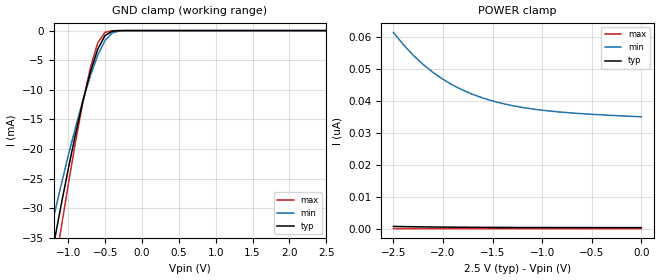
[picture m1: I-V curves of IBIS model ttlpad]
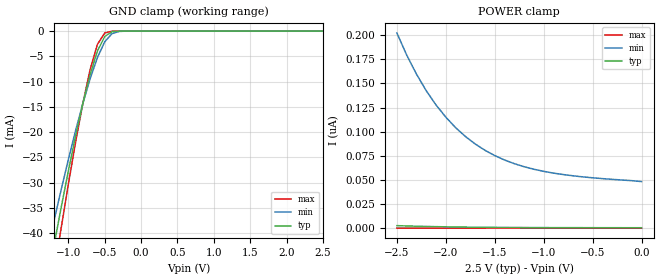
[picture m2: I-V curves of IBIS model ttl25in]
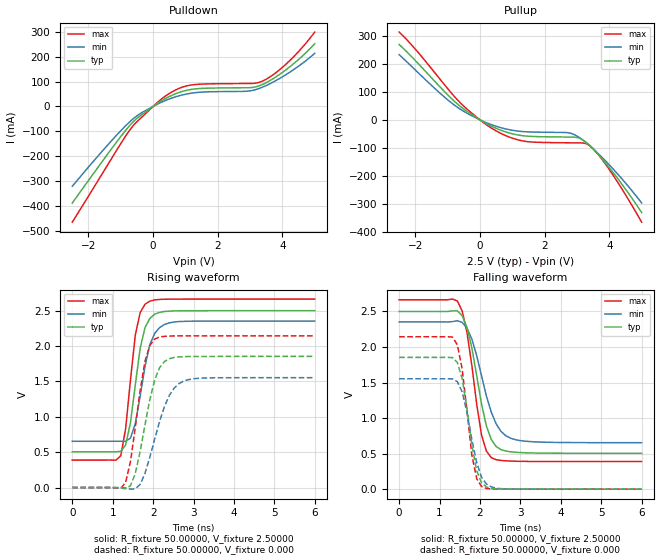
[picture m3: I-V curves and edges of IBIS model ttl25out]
| IBIS file idt45t9070.ibs created by s2ibis2 version 1.2
| North Carolina State University Electronics Research Laboratory  1995
[IBIS ver]   3.2
[File name]   idt45t9070.ibs
[File Rev]   1.0
[Date]   Friday, November 09, 2001
[Source]   Integrated Device Technology, Inc.
[Notes]
[Disclaimer] Integrated Device Technology, Inc. ("IDT") hereby grants the
   user of this IBIS model a non-exclusive, nontransferable
   license to use this IBIS model under the following terms. The
   user is granted this license only to use the IBIS model and is
   not granted rights to sell, copy (except as needed to run the
   IBIS model), rent, lease or sub-license the IBIS model in
   whole or in part, or in modified form to anyone. The User may
   modify the IBIS model to suit its specific applications, but
   rights to derivative works and such modifications shall belong
   to IDT. This IBIS model is provided on an AS IS" basis and IDT
   makes absolutely no warranty with respect to the information
   contained herein. IDT DISCLAIMS AND CUSTOMER WAIVES ALL
   WARRANTIES, EXPRESS AND IMPLIED, INCLUDING WARRANTIES OF
   MERCHANTABILITY AND FITNESS FOR A PARTICULAR PURPOSE. THE
   ENTIRE RISK AS TO QUALITY AND PERFORMANCE IS WITH THE USER
   ACCORDINGLY, IN NO EVENT SHALL IDT BE LIABLE FOR ANY DIRECT OR
   INDIRECT DAMAGES, WHETHER IN CONTRACT OR TORT, INCLUDING ANY
   LOST PROFITS OR OTHER INCIDENTAL, CONSEQUENTIAL, EXEMPLARY, OR
   PUNITIVE DAMAGES ARISING OUT OF THE USE OR APPLICATION OF THE
   IBIS model. Further, IDT reserves the right to make changes
   without notice to any product herein to improve reliability,
   function, or design. IDT does not convey any license under
   patent rights or any other intellectual property rights,
   including those of third parties. IDT is not obligated to
   provide maintenance or support for the licensed IBIS model.
[Copyright]   Copyright 2001, Integrated Device Technology, Inc. all rights
   reserved
|   Component idt45t9070
[Component]   idt45t9070
[Manufacturer]   Integrated Device Technology
|Package   PA48
[Package]
| variable   typ   min   max
R_pkg   6.00000m   6.00000m   6.00000m
L_pkg   3.00000nH   3.00000nH   3.00000nH
C_pkg   0.20000pF   0.20000pF   0.20000pF
[Pin]  signal_name   model_name   R_pin   L_pin   C_pin
1   gl   ttlpad
2   vdd   POWER
3   vdd   POWER
4   gnd   GND
5   gnd   GND
6   g1x   ttlpad
7   vddq   POWER
8   q2   ttl25out
9   q1   ttl25out
10   gnd   GND
11   vddq   POWER
12   gnd   GND
13   a   ttl25in
14   vddq   POWER
15   gnd   GND
16   q10   ttl25out
17   q9   ttl25out
18   vddq   POWER
19   g2x   ttlpad
20   gnd   GND
21   gnd   GND
22   vdd   POWER
23   vdd   POWER
24   NC   NC
25   NC   NC
26   gnd   GND
27   vddq   POWER
28   gnd   GND
29   gnd   GND
30   vddq   POWER
31   vddq   POWER
32   q8   ttl25out
33   q7   ttl25out
34   gnd   GND
35   vddq   POWER
36   q6   ttl25out
37   q5   ttl25out
38   vddq   POWER
39   gnd   GND
40   q4   ttl25out
41   q3   ttl25out
42   vddq   POWER
43   gnd   GND
44   gnd   GND
45   gnd   GND
46   vddq   POWER
47   vddq   POWER
48   gnd   GND
[Pin Mapping]  pulldown_ref   pullup_ref   gnd_clamp_ref   power_clamp_ref
1   gnd   vdd
2   NC   vdd
3   NC   vdd
4   gnd   NC
5   gnd   NC
6   gnd   vdd
7   NC   vddq
8   gnd   vddq
9   gnd   vddq
10   gnd   NC
11   NC   vddq
12   gnd   NC
13   gnd   vdd
14   NC   vddq
15   gnd   NC
16   gnd   vddq
17   gnd   vddq
18   NC   vddq
19   gnd   vdd
20   gnd   NC
21   gnd   NC
22   NC   vdd
23   NC   vdd
24   NC   NC
25   NC   NC
26   gnd   NC
27   NC   vddq
28   gnd   NC
29   gnd   NC
30   NC   vddq
31   NC   vddq
32   gnd   vddq
33   gnd   vddq
34   gnd   NC
35   NC   vddq
36   gnd   vddq
37   gnd   vddq
38   NC   vddq
39   gnd   NC
40   gnd   vddq
41   gnd   vddq
42   NC   vddq
43   gnd   NC
44   gnd   NC
45   gnd   NC
46   NC   vddq
47   NC   vddq
48   gnd   NC
| Models and submodels in the file (3): ttlpad (Input), ttl25in (Input), ttl25out (Output)
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|   Model ttlpad
[Model]   ttlpad
Model_type   Input
Polarity   Non-Inverting
Vinl =  0.70000V
Vinh =  1.70000V
Vmeas =  1.25000V
C_comp   5.00000pF   5.00000pF   5.00000pF
[Temperature Range]   45.00000   0.14000k   -30.00000
[Voltage Range]   2.50000V   2.30000V   2.70000V
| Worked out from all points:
|   GND clamp passes 1 mA (typ) near -0.51 V on its own axis
[GND_clamp]
| voltage   I(typ)   I(min)   I(max)
-2.5V     -129.2mA   -109.1mA   -150.6mA
-1.3V     -43.01mA   -37.08mA   -49.74mA
-1.2V     -36.24mA   -31.57mA   -41.59mA
-1.1V     -29.66mA   -26.23mA   -33.63mA
-900mV    -17.36mA   -16.23mA   -18.68mA
-800mV    -11.85mA   -11.7mA    -12mA
-700mV    -6.996mA   -7.615mA   -6.253mA
-600mV    -3.137mA   -4.151mA   -2.071mA
-500mV    -815.1uA   -1.634mA   -278.8uA
-400mV    -95.37uA   -373.7uA   -14.75uA
-300mV    -5.658uA   -48.78uA   -281.7nA
2.5V      324.7pA    35.28nA    828.2fA
[POWER_clamp]
| voltage   I(typ)   I(min)   I(max)
-2.5V     698.6pA    61.39nA    2.05pA
-2.4V     644.6pA    57.56nA    1.88pA
-2.3V     597.5pA    54.23nA    1.737pA
-2.2V     556.7pA    51.34nA    1.611pA
-2.1V     521.4pA    48.85nA    1.499pA
-1.9V     465pA      44.88nA    1.333pA
-1.8V     442.7pA    43.32nA    1.256pA
-1.6V     407.7pA    40.88nA    1.155pA
-1.3V     373.1pA    38.48nA    1.037pA
-1V       352.5pA    37.05nA    965.9fA
-600mV    337.2pA    35.97nA    899.5fA
0V        324.7pA    34.99nA    849.9fA
|   Model ttl25in
[Model]   ttl25in
Model_type   Input
Polarity   Non-Inverting
Vinl =  0.70000V
Vinh =  1.70000V
Vmeas =  1.25000V
C_comp   5.00000pF   5.00000pF   5.00000pF
[Temperature Range]   45.00000   0.14000k   -30.00000
[Voltage Range]   2.50000V   2.30000V   2.70000V
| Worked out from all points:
|   GND clamp passes 1 mA (typ) near -0.49 V on its own axis
[GND_clamp]
| voltage   I(typ)   I(min)   I(max)
-2.5V     -150.1mA   -128.5mA   -173mA
-1.3V     -50.47mA   -44.23mA   -57.51mA
-1.2V     -42.64mA   -37.76mA   -48.2mA
-1.1V     -35.02mA   -31.48mA   -39.1mA
-900mV    -20.73mA   -19.68mA   -21.96mA
-800mV    -14.28mA   -14.3mA    -14.26mA
-700mV    -8.553mA   -9.407mA   -7.567mA
-600mV    -3.939mA   -5.223mA   -2.609mA
-500mV    -1.074mA   -2.122mA   -375.8uA
-400mV    -131.3uA   -507.1uA   -20.31uA
-300mV    -7.825uA   -67.79uA   -384.6nA
2.5V      443.6pA    49.9nA     1.135pA
[POWER_clamp]
| voltage   I(typ)   I(min)   I(max)
-2.5V     2.616nA    202.4nA    8.153pA
-2.4V     2.294nA    179.5nA    7.17pA
-2.3V     2.014nA    159.7nA    6.305pA
-2.2V     1.772nA    142.5nA    5.573pA
-2.1V     1.564nA    127.7nA    4.925pA
-1.9V     1.231nA    104.2nA    3.911pA
-1.8V     1.1nA      95.05nA    3.496pA
-1.6V     895.6pA    80.73nA    2.854pA
-1.3V     696.3pA    66.86nA    2.22pA
-1V       581.4pA    58.89nA    1.825pA
-600mV    500.6pA    53.16nA    1.519pA
0V        443.6pA    48.28nA    1.265pA
|   Model ttl25out
[Model]   ttl25out
Model_type   Output
Polarity   Non-Inverting
Vmeas =  1.25000V
C_comp   5.00000pF   5.00000pF   5.00000pF
[Temperature Range]   45.00000   0.14000k   -30.00000
[Voltage Range]   2.50000V   2.30000V   2.70000V
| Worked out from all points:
|   slope of the pulldown table from 0 to 0.375 V, typ, clamps not added: 12.1 ohm
|   slope of the pullup table from 0 to 0.375 V, typ, clamps not added: 15.8 ohm
|   rising waveform, R_fixture 50.00000, V_fixture 2.50000: 20-80 % time 299ps typ, 329ps min, 257ps max; typ from 0.505 V to 2.5 V
|   rising waveform, R_fixture 50.00000, V_fixture 0.000: 20-80 % time 397ps typ, 498ps min, 324ps max; typ from 0 V to 1.85 V
|   falling waveform, R_fixture 50.00000, V_fixture 2.50000: 20-80 % time 402ps typ, 495ps min, 340ps max; typ from 2.5 V to 0.505 V
|   falling waveform, R_fixture 50.00000, V_fixture 0.000: 20-80 % time 302ps typ, 343ps min, 267ps max; typ from 1.85 V to 0 V
[Pulldown]
| voltage   I(typ)   I(min)   I(max)
-2.5V     -387.1mA   -320.1mA   -464mA
-1.3V     -172.3mA   -139.4mA   -211.9mA
-700mV    -73.11mA   -58.92mA   -90.86mA
-400mV    -37.65mA   -28.88mA   -48.96mA
300mV     25.63mA    19.24mA    33.79mA
700mV     51.07mA    38.83mA    66.42mA
1.1V      66.37mA    51.46mA    84.22mA
2.9V      74.99mA    61.06mA    92.02mA
3.4V      89.1mA     78.19mA    102.5mA
4.1V      145.9mA    126.7mA    168.2mA
4.5V      188.2mA    161.4mA    220mA
5V        251.4mA    212.9mA    298.1mA
[Pullup]
| voltage   I(typ)   I(min)   I(max)
-2.5V     269.9mA    233.5mA    314.3mA
-800mV    67.39mA    53.61mA    84.83mA
-300mV    22.62mA    17.64mA    28.64mA
400mV     -25.11mA   -19.06mA   -32.59mA
900mV     -46.72mA   -35.05mA   -61.28mA
1.4V      -57.66mA   -42.47mA   -76.9mA
2.8V      -61.54mA   -47.61mA   -82.16mA
3.1V      -66.62mA   -65.23mA   -82.46mA
3.4V      -92.17mA   -92.61mA   -92.89mA
3.7V      -128.7mA   -125.1mA   -129.7mA
4.1V      -185.6mA   -173.4mA   -194.7mA
5V        -331.7mA   -297.2mA   -366.3mA
[Ramp]
| variable   typ   min   max
dV/dt_r   1.11240/0.40582n   0.93180/0.51868n   1.28700/0.32381n
dV/dt_f   1.19718/0.40734n   1.02540/0.48502n   1.36524/0.35328n
R_load = 50.00000
[Rising Waveform]
R_fixture = 50.00000
V_fixture = 2.50000
C_fixture = 0.000F
R_dut = 6.00000m
L_dut = 3.00000nH
C_dut = 0.20000pF
| time   V(typ)   V(min)   V(max)
0s        504.9mV    653.9mV    388.5mV
1.2ns     511.8mV    654mV      449.4mV
1.32ns    600mV      653.5mV    831mV
1.44ns    916.8mV    698.2mV    1.52V
1.56ns    1.452V     905.6mV    2.158V
1.68ns    1.968V     1.29V      2.473V
1.8ns     2.263V     1.714V     2.592V
2.04ns    2.45V      2.18V      2.652V
2.4ns     2.494V     2.328V     2.663V
6ns       2.5V       2.353V     2.664V
[Rising Waveform]
R_fixture = 50.00000
V_fixture = 0.000
C_fixture = 0.000F
R_dut = 6.00000m
L_dut = 3.00000nH
C_dut = 0.20000pF
| time   V(typ)   V(min)   V(max)
0s        0V         0V         0V
1.2ns     -7.736mV   74.99uV    -11.29mV
1.32ns    -16.35mV   -5.463mV   72.34mV
1.44ns    25.8mV     -22.87mV   368.6mV
1.56ns    199.1mV    -17.97mV   853mV
1.8ns     889.2mV    201.3mV    1.786V
2.04ns    1.522V     686.6mV    2.099V
2.4ns     1.821V     1.301V     2.142V
2.76ns    1.85V      1.506V     2.144V
6ns       1.854V     1.553V     2.144V
[Falling Waveform]
R_fixture = 50.00000
V_fixture = 2.50000
C_fixture = 0.000F
R_dut = 6.00000m
L_dut = 3.00000nH
C_dut = 0.20000pF
| time   V(typ)   V(min)   V(max)
0s        2.5V       2.353V     2.664V
1.44ns    2.508V     2.37V      2.647V
1.56ns    2.442V     2.346V     2.506V
1.68ns    2.272V     2.263V     2.199V
1.8ns     1.984V     2.11V      1.734V
2.04ns    1.192V     1.591V     758.1mV
2.28ns    697.5mV    1.083V     443mV
2.52ns    556.5mV    813.2mV    404mV
2.88ns    519mV      695.7mV    393.1mV
6ns       504.9mV    654mV      388.5mV
[Falling Waveform]
R_fixture = 50.00000
V_fixture = 0.000
C_fixture = 0.000F
R_dut = 6.00000m
L_dut = 3.00000nH
C_dut = 0.20000pF
| time   V(typ)   V(min)   V(max)
0s        1.854V     1.553V     2.144V
1.32ns    1.851V     1.552V     2.14V
1.44ns    1.783V     1.512V     2.031V
1.56ns    1.554V     1.367V     1.687V
1.8ns     618.1mV    696.3mV    476.7mV
1.92ns    255.7mV    369mV      145.9mV
2.04ns    90.47mV    165.6mV    37.04mV
2.28ns    10.07mV    32.31mV    3.092mV
2.52ns    2.521mV    7.211mV    1.099mV
6ns       941.7nV    3.235uV    0V
